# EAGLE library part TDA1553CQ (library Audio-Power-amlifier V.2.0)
The TDA1553CQ is a monolithic integrated class-B output amplifier in a 13-lead plastic DIL-bent-SIL power package. It contains 2 ´ 22 W amplifiers in BTL configuration.
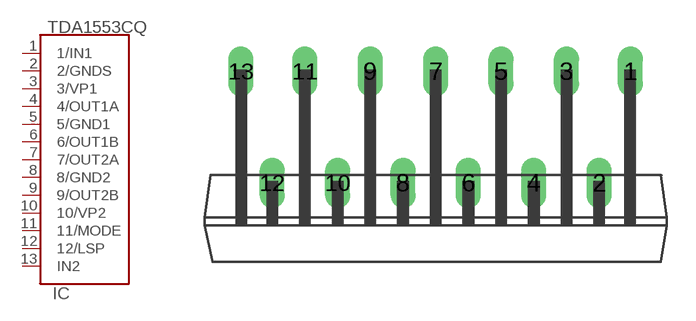
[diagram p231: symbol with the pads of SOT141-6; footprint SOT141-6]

Designator prefix IC

## TDA1553CQ  [SOT141-6]
1  1/IN1  in
2  2/GNDS  pwr
3  3/VP1  pwr
4  4/OUT1A  out
5  5/GND1  pwr
6  6/OUT1B  out
7  7/OUT2A  out
8  8/GND2  pwr
9  9/OUT2B  out
10  10/VP2  pwr
11  11/MODE  in
12  12/LSP
13  IN2  in

## Footprint SOT141-6 (pad centres in mm)
drill 0.8 long: 1 10.12,5.8; 2 8.5,0; 3 6.8,5.8; 4 5.1,0; 5 3.4,5.8; 6 1.7,0; 7 0,5.8; 8 -1.7,0; 9 -3.4,5.8; 10 -5.1,0; 11 -6.8,5.8; 12 -8.5,0; 13 -10.12,5.8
